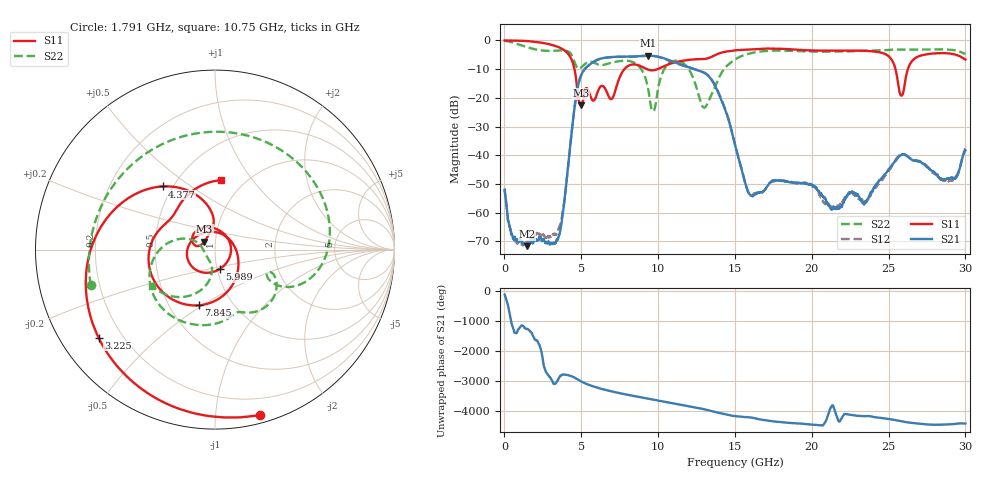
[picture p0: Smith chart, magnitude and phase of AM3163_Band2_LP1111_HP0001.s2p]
!Agilent Technologies,E8364B,MY43040894,A.07.50.67
!Agilent E8364B: A.07.50.67
!Date: Thursday, August 20, 2020 12:06:40
!Correction: S11(Full 2 Port(1,2))
!S21(Full 2 Port(1,2))
!S12(Full 2 Port(1,2))
!S22(Full 2 Port(1,2))
!S2P File: Measurements: S11, S21, S12, S22:
# Hz S  dB  R 50
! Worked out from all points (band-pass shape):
!   3201 points, 10 MHz to 30 GHz, reference 50 ohm
!   highest |S21| = -5.35 dB at 9.373 GHz (marker M1); lowest = -71.7 dB at 1.472 GHz (marker M2)
!   |S21| within 3 dB of the highest: 5.568 GHz to 11.45 GHz (5.884 GHz wide, 69.1 % of centre)
!   lowest |S11| = -22.6 dB at 4.986 GHz (marker M3), VSWR 1.16, Z = 44.2 + j4 ohm
!   |S11| at or under -10 dB: 4.556 GHz to 7.813 GHz (3.257 GHz wide, 52.7 % of centre); 9.265 GHz to 9.981 GHz (716.2 MHz wide, 7.44 % of centre); 25.45 GHz to 26.26 GHz (806.8 MHz wide, 3.12 % of centre)
!   |S22| runs from -24.7 to -0.2 dB; largest |S21 - S12| = 0.013
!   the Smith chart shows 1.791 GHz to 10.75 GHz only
!   S11 on the Smith chart (normalised r, x): 1.791 GHz: 0.06, -1.30; 3.225 GHz: 0.11, -0.33; 4.377 GHz: 0.44, +0.39; 5.989 GHz: 1.03, -0.22; 7.845 GHz: 0.70, -0.48; 10.75 GHz: 0.78, +0.72
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1e7  -0.04 -3.0  -52.29 -119.3  -51.54 119.8  -0.16 -6.8
1.472012e9  -0.26 -61.2  -71.66 175.6  -70.33 -46.4  -2.37 -137.4
1.790656e9  -0.41 -74.9  -69.86 30.5  -69.05 -69.2  -2.85 -164.1
3.224553e9  -1.79 -142.9  -70.82 150.8  -67.44 -8.2  -3.64 82.7
4.377294e9  -6.79 129.7  -31.87 44.1  -31.87 43.9  -5.18 -17.4
4.986466e9  -22.59 142.8  -12.19 -125.4  -12.19 -125.7  -9.52 -22.0
5.014581e9  -22.53 148.1  -11.84 -133.2  -11.84 -133.4  -9.37 -22.1
5.989256e9  -19.16 -75.2  -6.91 34.6  -6.94 34.5  -8.17 -63.9
6.888956e9  -20.36 80.5  -5.83 -88.7  -5.89 -88.9  -7.86 -85.1
7.844888e9  -9.81 -106.3  -5.66 165.5  -5.70 165.8  -7.09 -121.5
9.372503e9  -10.22 150.7  -5.35 17.4  -5.33 17.3  -17.46 156.8
1.000979e10  -9.93 128.1  -5.71 -45.3  -5.74 -46.0  -16.37 -98.6
1.075017e10  -8.20 84.9  -6.95 -115.8  -7.17 -116.1  -7.84 -149.9
1.300879e10  -6.48 -50.4  -11.32 27.2  -11.26 28.7  -23.42 -102.5
1.5005e10  -3.49 -133.0  -36.37 159.7  -36.33 158.8  -6.69 -112.2
1.598905e10  -3.17 -173.9  -53.75 116.3  -54.03 117.3  -4.54 -171.6
1.786342e10  -2.89 98.2  -48.80 -37.2  -48.74 -36.2  -3.58 92.3
2.000958e10  -3.52 -10.2  -50.36 -120.9  -50.74 -121.1  -3.93 -9.8
2.230569e10  -3.57 -100.0  -53.88 -138.1  -54.07 -133.1  -3.85 -93.6
2.500479e10  -5.54 158.2  -44.94 64.4  -45.48 64.4  -3.37 -167.8
2.583889e10  -19.25 171.3  -39.84 -11.7  -39.76 -9.7  -3.22 169.5
3e10  -6.68 50.8  -38.38 -88.1  -37.60 -86.0  -4.76 54.6
